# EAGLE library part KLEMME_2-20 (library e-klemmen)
Klemme 2 20
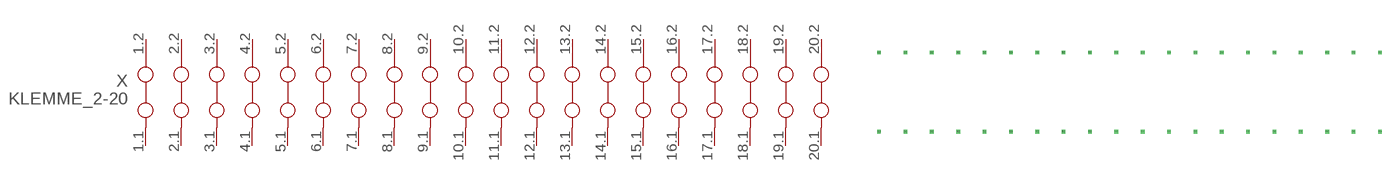
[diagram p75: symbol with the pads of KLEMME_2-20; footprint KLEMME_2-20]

Designator prefix X

## KLEMME_2-20  [KLEMME_2-20]
1.1  1.1  pas
1.2  1.2  pas
2.1  2.1  pas
2.2  2.2  pas
3.1  3.1  pas
3.2  3.2  pas
4.1  4.1  pas
4.2  4.2  pas
5.1  5.1  pas
5.2  5.2  pas
6.1  6.1  pas
6.2  6.2  pas
7.1  7.1  pas
7.2  7.2  pas
8.1  8.1  pas
8.2  8.2  pas
9.1  9.1  pas
9.2  9.2  pas
10.1  10.1  pas
10.2  10.2  pas
11.1  11.1  pas
11.2  11.2  pas
12.1  12.1  pas
12.2  12.2  pas
13.1  13.1  pas
13.2  13.2  pas
14.1  14.1  pas
14.2  14.2  pas
15.1  15.1  pas
15.2  15.2  pas
16.1  16.1  pas
16.2  16.2  pas
17.1  17.1  pas
17.2  17.2  pas
18.1  18.1  pas
18.2  18.2  pas
19.1  19.1  pas
19.2  19.2  pas
20.1  20.1  pas
20.2  20.2  pas

## Footprint KLEMME_2-20 (pad centres in mm)
Dummy
drill 0.2 pad 0.6 square: 1.1 0,-7.62; 1.2 0,7.62; 2.1 5.08,-7.62; 2.2 5.08,7.62; 3.1 10.16,-7.62; 3.2 10.16,7.62; 4.1 15.24,-7.62; 4.2 15.24,7.62; 5.1 20.32,-7.62; 5.2 20.32,7.62; 6.1 25.4,-7.62; 6.2 25.4,7.62; 7.1 30.48,-7.62; 7.2 30.48,7.62; 8.1 35.56,-7.62; 8.2 35.56,7.62; 9.1 40.64,-7.62; 9.2 40.64,7.62; 10.1 45.72,-7.62; 10.2 45.72,7.62; 11.1 50.8,-7.62; 11.2 50.8,7.62; 12.1 55.88,-7.62; 12.2 55.88,7.62; 13.1 60.96,-7.62; 13.2 60.96,7.62; 14.1 66.04,-7.62; 14.2 66.04,7.62; 15.1 71.12,-7.62; 15.2 71.12,7.62; 16.1 76.2,-7.62; 16.2 76.2,7.62; 17.1 81.28,-7.62; 17.2 81.28,7.62; 18.1 86.36,-7.62; 18.2 86.36,7.62; 19.1 91.44,-7.62; 19.2 91.44,7.62; 20.1 96.52,-7.62; 20.2 96.52,7.62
